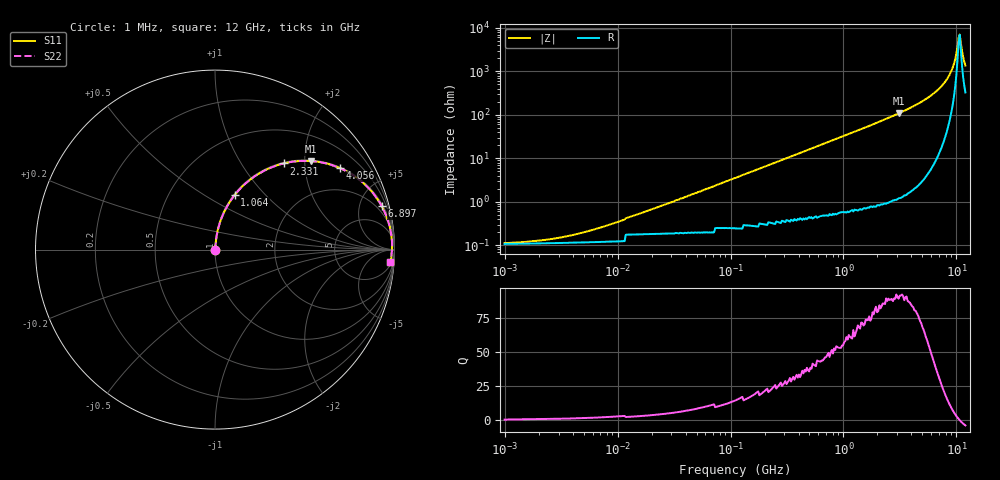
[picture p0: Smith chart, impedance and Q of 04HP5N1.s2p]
# MHz S MA R 50
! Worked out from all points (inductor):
!   408 points, 1 MHz to 12 GHz, reference 50 ohm
!   read as one part in series: L = 5.1 nH near 17.09 MHz
!   highest Q = 91.2 at 3.075 GHz (marker M1), where L = 5.57 nH
!   self-resonance near 10.45 GHz
!   S11 on the Smith chart (normalised r, x): 1 MHz: 1.00, +0.00; 1.064 GHz: 1.01, +0.69; 2.331 GHz: 1.02, +1.57; 4.056 GHz: 1.04, +3.04; 6.897 GHz: 1.24, +7.63; 12 GHz: 8, -27
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1  0.001188 15.6  0.999 -0.0  0.999 -0.0  0.001188 15.6
2.349  0.001434 31.6  0.999 -0.0  0.999 -0.0  0.001434 31.6
4.803  0.002024 49.3  0.999 -0.1  0.999 -0.1  0.002024 49.3
23.071  0.007572 76.7  0.998 -0.4  0.998 -0.4  0.007572 76.7
110.816  0.035 83.9  0.997 -2.0  0.997 -2.0  0.035 83.9
532.275  0.168 78.9  0.982 -9.7  0.982 -9.7  0.168 78.9
1063.684  0.324 70.1  0.941 -18.9  0.941 -18.9  0.324 70.1
1611.457  0.465 61.5  0.879 -27.7  0.879 -27.7  0.465 61.5
2331.2  0.614 51.5  0.782 -37.9  0.782 -37.9  0.614 51.5
2556.642  0.653 48.6  0.75 -40.7  0.75 -40.7  0.653 48.6
3075.037  0.728 42.6  0.677 -46.7  0.677 -46.7  0.728 42.6
4056.215  0.831 33.1  0.546 -56.2  0.546 -56.2  0.831 33.1
5475.38  0.917 22.6  0.384 -66.5  0.384 -66.5  0.917 22.6
6896.676  0.96 14.6  0.252 -73.7  0.252 -73.7  0.96 14.6
7920.912  0.976 9.8  0.171 -77.1  0.171 -77.1  0.976 9.8
8889.718  0.984 6.0  0.104 -78.2  0.104 -78.2  0.984 6.0
9526.989  0.986 3.7  0.065 -75.9  0.065 -75.9  0.986 3.7
10209.94  0.987 1.4  0.027 -59.5  0.027 -59.5  0.987 1.4
10448.31  0.986 0.6  0.017 -36.3  0.017 -36.3  0.986 0.6
10941.86  0.985 -0.9  0.022 47.2  0.022 47.2  0.985 -0.9
11458.72  0.983 -2.5  0.046 67.2  0.046 67.2  0.983 -2.5
12000  0.98 -4.0  0.072 72.1  0.072 72.1  0.98 -4.0
